(* Logix 5000 AddOnInstructionDefinition export ME_AOI_546xx_E02; software revision 20.05 *)

TYPE ME_IOL_PORT_32B :   // 32 Reserved IOL Bytes for IN & OUT
STRUCT
   in_data : SINT[32];
   out_data : SINT[32];
END_STRUCT
END_TYPE

TYPE ME_UDT_546xx_E02_In :   // 546xx Input Assembly
STRUCT
   Digital_Inputs : SINT[2];
   DI_Qualifier : SINT[2];
   DO_Qualifier : SINT[2];
   System_Status : ME_546xx_System_Status;
   Diagnostic_1 : ME_Diag_546xx;
   Diagnostic_2 : ME_Diag_546xx;
   Diagnostic_3 : ME_Diag_546xx;
   Diagnostic_4 : ME_Diag_546xx;
   Diagnostic_5 : ME_Diag_546xx;
   Diagnostic_6 : ME_Diag_546xx;
   Diagnostic_7 : ME_Diag_546xx;
   Diagnostic_8 : ME_Diag_546xx;
   IOL_PortX0_Status : ME_IOL_Port_X_Status_546xx;
   IOL_PortX1_Status : ME_IOL_Port_X_Status_546xx;
   IOL_PortX2_Status : ME_IOL_Port_X_Status_546xx;
   IOL_PortX3_Status : ME_IOL_Port_X_Status_546xx;
   IOL_PortX4_Status : ME_IOL_Port_X_Status_546xx;
   IOL_PortX5_Status : ME_IOL_Port_X_Status_546xx;
   IOL_PortX6_Status : ME_IOL_Port_X_Status_546xx;
   IOL_PortX7_Status : ME_IOL_Port_X_Status_546xx;
END_STRUCT
END_TYPE

TYPE ME_546xx_System_Status :   // Block Diagnostic Status
STRUCT
   Under_Voltage_Bus_Sensor_Supply : BOOL;
   Under_Voltage_Actuator_Supply : BOOL;
   No_Actuator_Supply : BOOL;
   External_Error : BOOL;
   Channel_Has_A_Sensor_Short_Circuit : BOOL;
   Channel_Has_An_Actuator_Short_Circuit : BOOL;
   Channel_Has_An_Actuator_Warning : BOOL;
   At_Least_One_Analog_Channel_Has_An_Error : BOOL;
   Internal_Communication_Error : BOOL;
   At_Least_One_IO_Link_Channel_Has_an_Erro : BOOL;
   Over_Voltage_Bus_Sensor_Supply : BOOL;
   Over_Voltage_Actuator_ASupply : BOOL;
   IO_Link_Channel_Has_A_Wire_Break : BOOL;
END_STRUCT
END_TYPE

TYPE ME_UDT_546xx_E02_Out :   // 546xx Output Assembly
STRUCT
   Digital_Outputs : SINT[2];
   Acknowledge : SINT[2];
END_STRUCT
END_TYPE

TYPE ME_Diag_546xx :   // Diagnostic Buffer for 546xx Modules
STRUCT
   IP : SINT;   // Last Octet of IP
   Identification : SINT;   // 0 = Default, 40h = IOL Master, 41h = IOL Device, 42h = Murr IOLD
   Channel_number : SINT;   // Digital Diag = Pin/Port IOL Diag = IOL Channel
   Error_Code_1 : SINT;   // Global Error Code or IOL LSB
   Error_Code_2 : SINT;   // Specific Error Code or IOL MSB
   Status : BOOL;   // 0 = Inactive, 1 = Active
   Severity : SINT;   // 1 = Minor, 2 = Major, 3 = Info
   Count : SINT;
END_STRUCT
END_TYPE

TYPE ME_UDT_546xx_E02 :   // Setup for EDS - E02 DIO + STATUS + DIAG
STRUCT
   I : ME_UDT_546xx_E02_In;
   O : ME_UDT_546xx_E02_Out;
END_STRUCT
END_TYPE

TYPE ME_IOL_Port_X_Status_546xx :   // Status of the IO-Link Device
STRUCT
   DevCom : BOOL;   // Pre-Operate or Operate Mode
   DevErr : BOOL;   // IOL Device Error or Warning
   PQ : BOOL;   // Valid Process Data Exchanged between Device & Master
   IOLD_Vendor_ID : SINT[2];   // Vendor ID of IO-Link Device
   IOLD_Device_ID : SINT[4];   // Device IP of IO-Link Device
END_STRUCT
END_TYPE

ADD_ON_INSTRUCTION ME_AOI_546xx_E02   (* revision 0.1 *)
VAR_IN_OUT
   Raw_546xx_Input : SINT[394]; {required}
   Raw_546xx_Output : SINT[259]; {required}
   Mapped_546xx_Communication_Data : ME_UDT_546xx_E02; {required}
   IO_Link_Port_X0 : ME_IOL_PORT_32B; {required}
        .I.DATA.0   // Input Port 0 Pin 4
        .I.DATA.1   // Input Port 0 Pin 2
        .I.DATA.2   // Input Port 1 Pin 4
        .I.DATA.3   // Input Port 1 Pin 2
        .I.DATA.4   // Input Port 2 Pin 4
        .I.DATA.5   // Input Port 2 Pin 2
        .I.DATA.6   // Input Port 3 Pin 4
        .I.DATA.7   // Input Port 3 Pin 2
        .I.DATA.8   // Input Port 4 Pin 4
        .I.DATA.9   // Input Port 4 Pin 2
        .I.DATA.10   // Input Port 5 Pin 4
        .I.DATA.11   // Input Port 5 Pin 2
        .I.DATA.12   // Input Port 6 Pin 4
        .I.DATA.13   // Input Port 6 Pin 2
        .I.DATA.14   // Input Port 7 Pin 4
        .I.DATA.15   // Input Port 7 Pin 2
        .I.OVERLOAD.0   // Port 0 Pin 4 Output Overload Status
        .I.OVERLOAD.1   // Port 0 Pin 2 Output Overload Status
        .I.OVERLOAD.2   // Port 1 Pin 4 Output Overload Status
        .I.OVERLOAD.3   // Port 1 Pin 2 Output Overload Status
        .I.OVERLOAD.4   // Port 2 Pin 4 Output Overload Status
        .I.OVERLOAD.5   // Port 2 Pin 2 Output Overload Status
        .I.OVERLOAD.6   // Port 3 Pin 4 Output Overload Status
        .I.OVERLOAD.7   // Port 3 Pin 2 Output Overload Status
        .I.OVERLOAD.8   // Port 4 Pin 4 Output Overload Status
        .I.OVERLOAD.9   // Port 4 Pin 2 Output Overload Status
        .I.OVERLOAD.10   // Port 5 Pin 4 Output Overload Status
        .I.OVERLOAD.11   // Port 5 Pin 2 Output Overload Status
        .I.OVERLOAD.12   // Port 6 Pin 4 Output Overload Status
        .I.OVERLOAD.13   // Port 6 Pin 2 Output Overload Status
        .I.OVERLOAD.14   // Port 7 Pin 4 Output Overload Status
        .I.OVERLOAD.15   // Port 7 Pin 2 Output Overload Status
        .I.PORT_1_DEVICE_CONNECTED   // Port 1 I/O Link Device Connected
        .I.PORT_1_IO_LINK_STATUS   // Port 1 In I/O Link Mode
        .I.PORT_1_VALIDATION_FAILED   // Port 1 I/O Link Device Configuration Mismatch
        .I.PORT_2_DEVICE_CONNECTED   // Port 2 I/O Link Device Connected
        .I.PORT_2_IO_LINK_STATUS   // Port 2 In I/O Link Mode
        .I.PORT_2_VALIDATION_FAILED   // Port 2 I/O Link Device Configuration Mismatch
        .I.PORT_3_DEVICE_CONNECTED   // Port 3 I/O Link Device Connected
        .I.PORT_3_IO_LINK_STATUS   // Port 3 In I/O Link Mode
        .I.PORT_3_VALIDATION_FAILED   // Port 3 I/O Link Device Configuration Mismatch
        .I.PORT_4_DEVICE_CONNECTED   // Port 4 I/O Link Device Connected
        .I.PORT_4_IO_LINK_STATUS   // Port 4 In I/O Link Mode
        .I.PORT_4_VALIDATION_FAILED   // Port 4 I/O Link Device Configuration Mismatch
        .I.SHORT_CIRCUIT.0   // Port 0 Pin 4 Short Circuit
        .I.SHORT_CIRCUIT.1   // Port 0 Pin 2 Short Circuit
        .I.SHORT_CIRCUIT.2   // Port 1 Pin 4 Short Circuit
        .I.SHORT_CIRCUIT.3   // Port 1 Pin 2 Short Circuit
        .I.SHORT_CIRCUIT.4   // Port 2 Pin 4 Short Circuit
        .I.SHORT_CIRCUIT.5   // Port 2 Pin 2 Short Circuit
        .I.SHORT_CIRCUIT.6   // Port 3 Pin 4 Short Circuit
        .I.SHORT_CIRCUIT.7   // Port 3 Pin 2 Short Circuit
        .I.SHORT_CIRCUIT.8   // Port 4 Pin 4 Short Circuit
        .I.SHORT_CIRCUIT.9   // Port 4 Pin 2 Short Circuit
        .I.SHORT_CIRCUIT.10   // Port 5 Pin 4 Short Circuit
        .I.SHORT_CIRCUIT.11   // Port 5 Pin 2 Short Circuit
        .I.SHORT_CIRCUIT.12   // Port 6 Pin 4 Short Circuit
        .I.SHORT_CIRCUIT.13   // Port 6 Pin 2 Short Circuit
        .I.SHORT_CIRCUIT.14   // Port 7 Pin 4 Short Circuit
        .I.SHORT_CIRCUIT.15   // Port 7 Pin 2 Short Circuit
        .I.UA_FAULT   // Output Power from Aux Power cable Under Voltage
        .I.US_FAULT   // Module Power from IO-Link Communication Cable Under Voltage
        .O.DATA.0   // Output Port 0 Pin 4
        .O.DATA.1   // Output Port 0 Pin 2
        .O.DATA.2   // Output Port 1 Pin 4
        .O.DATA.3   // Output Port 1 Pin 2
        .O.DATA.4   // Output Port 2 Pin 4
        .O.DATA.5   // Output Port 2 Pin 2
        .O.DATA.6   // Output Port 3 Pin 4
        .O.DATA.7   // Output Port 3 Pin 2
        .O.DATA.8   // Output Port 4 Pin 4
        .O.DATA.9   // Output Port 4 Pin 2
        .O.DATA.10   // Output Port 5 Pin 4
        .O.DATA.11   // Output Port 5 Pin 2
        .O.DATA.12   // Output Port 6 Pin 4
        .O.DATA.13   // Output Port 6 Pin 2
        .O.DATA.14   // Output Port 7 Pin 4
        .O.DATA.15   // Output Port 7 Pin 2
        .O.DISPLAY_GREEN   // Green LED On
        .O.DISPLAY_LOCK   // Display Lock PLC Lock
        .O.DISPLAY_RED   // Red LED On
        .O.RESTART.0   // Port 0 Pin 4 Output Restart
        .O.RESTART.1   // Port 0 Pin 2 Output Restart
        .O.RESTART.2   // Port 1 Pin 4 Output Restart
        .O.RESTART.3   // Port 1 Pin 2 Output Restart
        .O.RESTART.4   // Port 2 Pin 4 Output Restart
        .O.RESTART.5   // Port 2 Pin 2 Output Restart
        .O.RESTART.6   // Port 3 Pin 4 Output Restart
        .O.RESTART.7   // Port 3 Pin 2 Output Restart
        .O.RESTART.8   // Port 4 Pin 4 Output Restart
        .O.RESTART.9   // Port 4 Pin 2 Output Restart
        .O.RESTART.10   // Port 5 Pin 4 Output Restart
        .O.RESTART.11   // Port 5 Pin 2 Output Restart
        .O.RESTART.12   // Port 6 Pin 4 Output Restart
        .O.RESTART.13   // Port 6 Pin 2 Output Restart
        .O.RESTART.14   // Port 7 Pin 4 Output Restart
        .O.RESTART.15   // Port 7 Pin 2 Output Restart
   IO_Link_Port_X1 : ME_IOL_PORT_32B; {required}
   IO_Link_Port_X2 : ME_IOL_PORT_32B; {required}
   IO_Link_Port_X3 : ME_IOL_PORT_32B; {required}
   IO_Link_Port_X4 : ME_IOL_PORT_32B; {required}
   IO_Link_Port_X5 : ME_IOL_PORT_32B; {required}
   IO_Link_Port_X6 : ME_IOL_PORT_32B; {required}
   IO_Link_Port_X7 : ME_IOL_PORT_32B; {required}
END_VAR

ROUTINE Logic   (* ladder *)
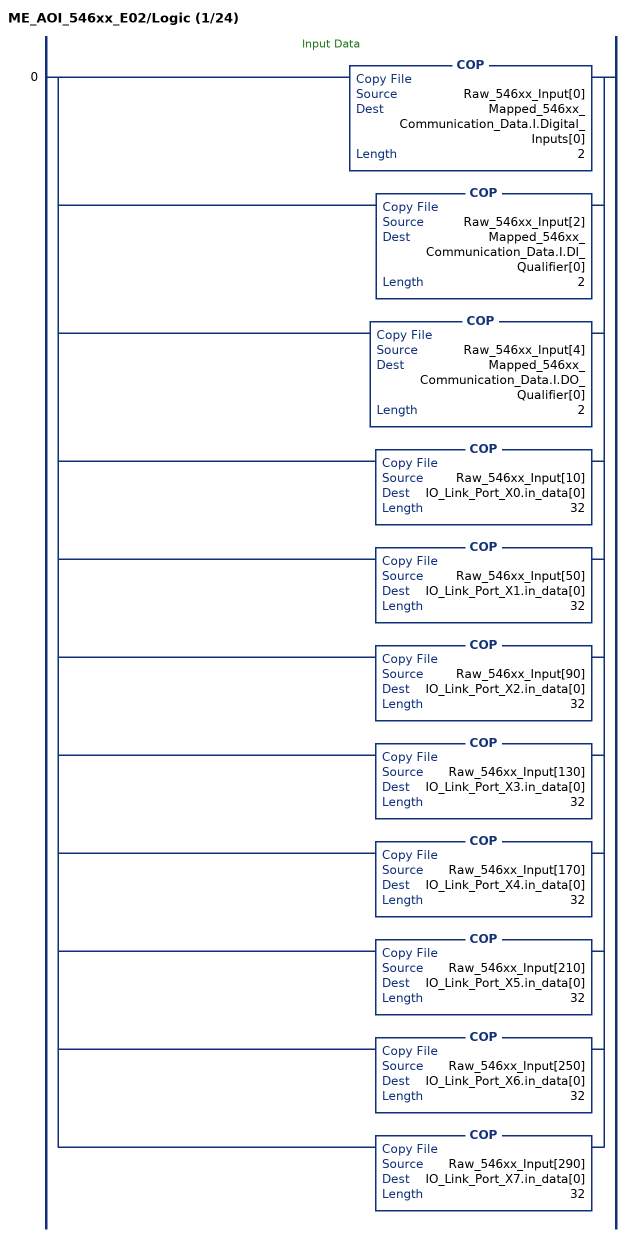
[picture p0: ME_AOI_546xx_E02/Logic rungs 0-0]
   // Input Data
   0: [COP(Raw_546xx_Input[0],Mapped_546xx_Communication_Data.I.Digital_Inputs[0],2) ,COP(Raw_546xx_Input[2],Mapped_546xx_Communication_Data.I.DI_Qualifier[0],2) ,COP(Raw_546xx_Input[4],Mapped_546xx_Communication_Data.I.DO_Qualifier[0],2) ,COP(Raw_546xx_Input[10],IO_Link_Port_X0.in_data[0],32) ,COP(Raw_546xx_Input[50],IO_Link_Port_X1.in_data[0],32) ,COP(Raw_546xx_Input[90],IO_Link_Port_X2.in_data[0],32) ,COP(Raw_546xx_Input[130],IO_Link_Port_X3.in_data[0],32) ,COP(Raw_546xx_Input[170],IO_Link_Port_X4.in_data[0],32) ,COP(Raw_546xx_Input[210],IO_Link_Port_X5.in_data[0],32) ,COP(Raw_546xx_Input[250],IO_Link_Port_X6.in_data[0],32) ,COP(Raw_546xx_Input[290],IO_Link_Port_X7.in_data[0],32) ];
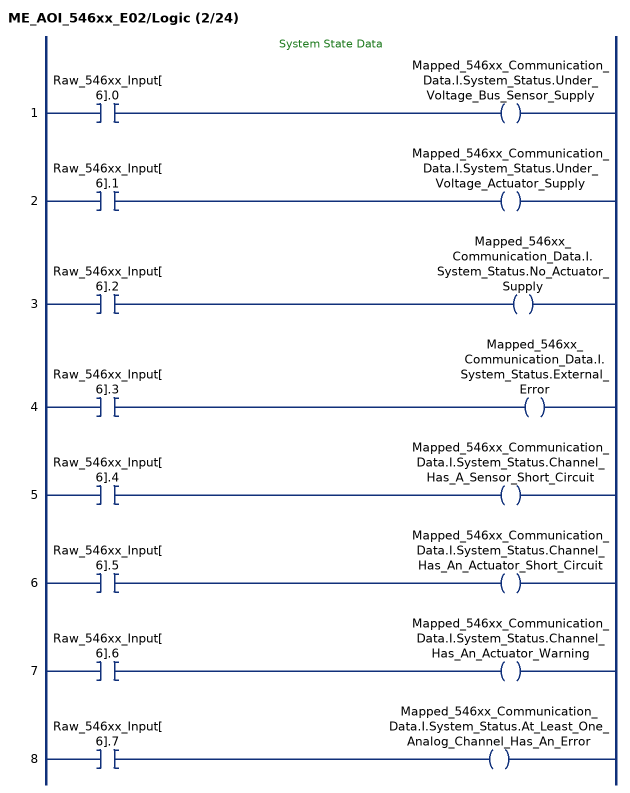
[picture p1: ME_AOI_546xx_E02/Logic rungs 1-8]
   // System State Data
   1: XIC(Raw_546xx_Input[6].0)OTE(Mapped_546xx_Communication_Data.I.System_Status.Under_Voltage_Bus_Sensor_Supply);
   2: XIC(Raw_546xx_Input[6].1)OTE(Mapped_546xx_Communication_Data.I.System_Status.Under_Voltage_Actuator_Supply);
   3: XIC(Raw_546xx_Input[6].2)OTE(Mapped_546xx_Communication_Data.I.System_Status.No_Actuator_Supply);
   4: XIC(Raw_546xx_Input[6].3)OTE(Mapped_546xx_Communication_Data.I.System_Status.External_Error);
   5: XIC(Raw_546xx_Input[6].4)OTE(Mapped_546xx_Communication_Data.I.System_Status.Channel_Has_A_Sensor_Short_Circuit);
   6: XIC(Raw_546xx_Input[6].5)OTE(Mapped_546xx_Communication_Data.I.System_Status.Channel_Has_An_Actuator_Short_Circuit);
   7: XIC(Raw_546xx_Input[6].6)OTE(Mapped_546xx_Communication_Data.I.System_Status.Channel_Has_An_Actuator_Warning);
   8: XIC(Raw_546xx_Input[6].7)OTE(Mapped_546xx_Communication_Data.I.System_Status.At_Least_One_Analog_Channel_Has_An_Error);
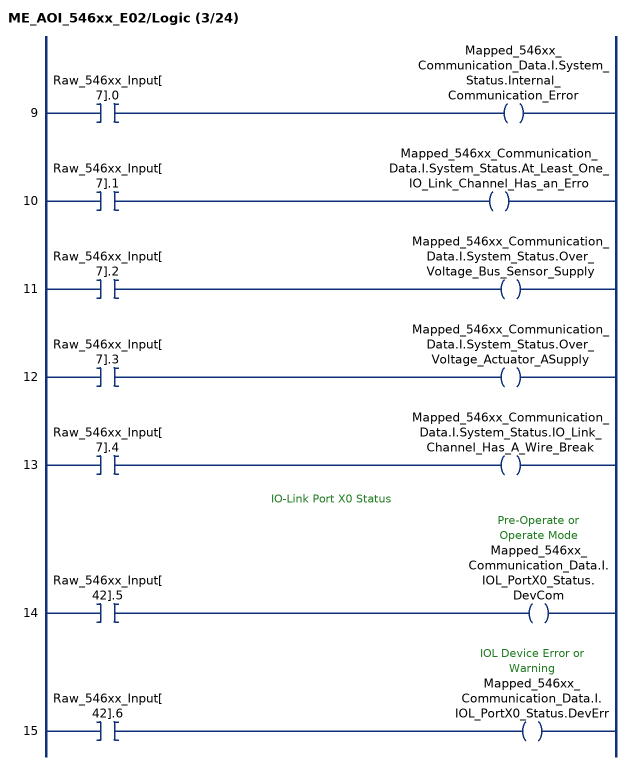
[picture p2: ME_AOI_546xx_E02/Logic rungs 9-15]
   9: XIC(Raw_546xx_Input[7].0)OTE(Mapped_546xx_Communication_Data.I.System_Status.Internal_Communication_Error);
   10: XIC(Raw_546xx_Input[7].1)OTE(Mapped_546xx_Communication_Data.I.System_Status.At_Least_One_IO_Link_Channel_Has_an_Erro);
   11: XIC(Raw_546xx_Input[7].2)OTE(Mapped_546xx_Communication_Data.I.System_Status.Over_Voltage_Bus_Sensor_Supply);
   12: XIC(Raw_546xx_Input[7].3)OTE(Mapped_546xx_Communication_Data.I.System_Status.Over_Voltage_Actuator_ASupply);
   13: XIC(Raw_546xx_Input[7].4)OTE(Mapped_546xx_Communication_Data.I.System_Status.IO_Link_Channel_Has_A_Wire_Break);
   // IO-Link Port X0 Status
   14: XIC(Raw_546xx_Input[42].5)OTE(Mapped_546xx_Communication_Data.I.IOL_PortX0_Status.DevCom);
   15: XIC(Raw_546xx_Input[42].6)OTE(Mapped_546xx_Communication_Data.I.IOL_PortX0_Status.DevErr);
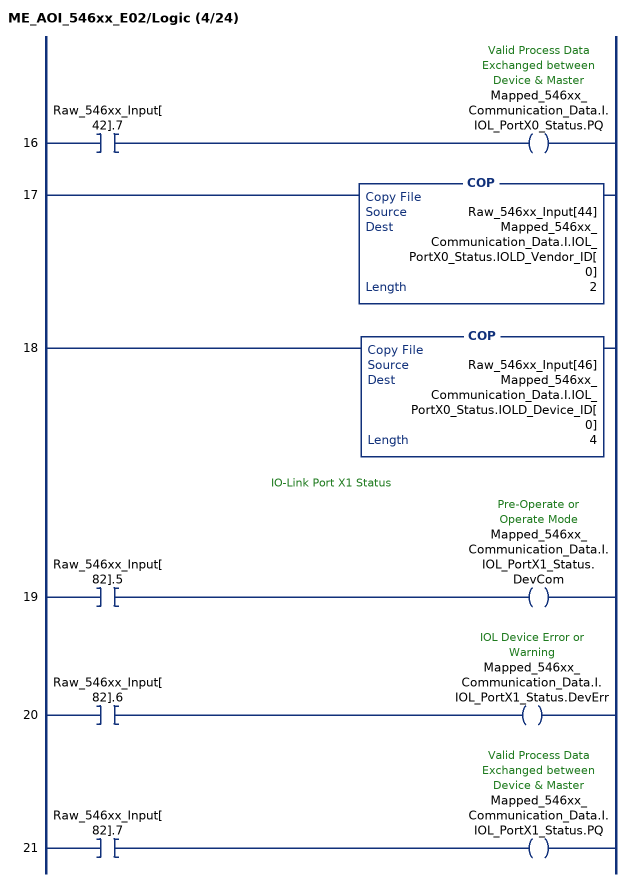
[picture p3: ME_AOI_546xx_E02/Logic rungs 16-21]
   16: XIC(Raw_546xx_Input[42].7)OTE(Mapped_546xx_Communication_Data.I.IOL_PortX0_Status.PQ);
   17: COP(Raw_546xx_Input[44],Mapped_546xx_Communication_Data.I.IOL_PortX0_Status.IOLD_Vendor_ID[0],2);
   18: COP(Raw_546xx_Input[46],Mapped_546xx_Communication_Data.I.IOL_PortX0_Status.IOLD_Device_ID[0],4);
   // IO-Link Port X1 Status
   19: XIC(Raw_546xx_Input[82].5)OTE(Mapped_546xx_Communication_Data.I.IOL_PortX1_Status.DevCom);
   20: XIC(Raw_546xx_Input[82].6)OTE(Mapped_546xx_Communication_Data.I.IOL_PortX1_Status.DevErr);
   21: XIC(Raw_546xx_Input[82].7)OTE(Mapped_546xx_Communication_Data.I.IOL_PortX1_Status.PQ);
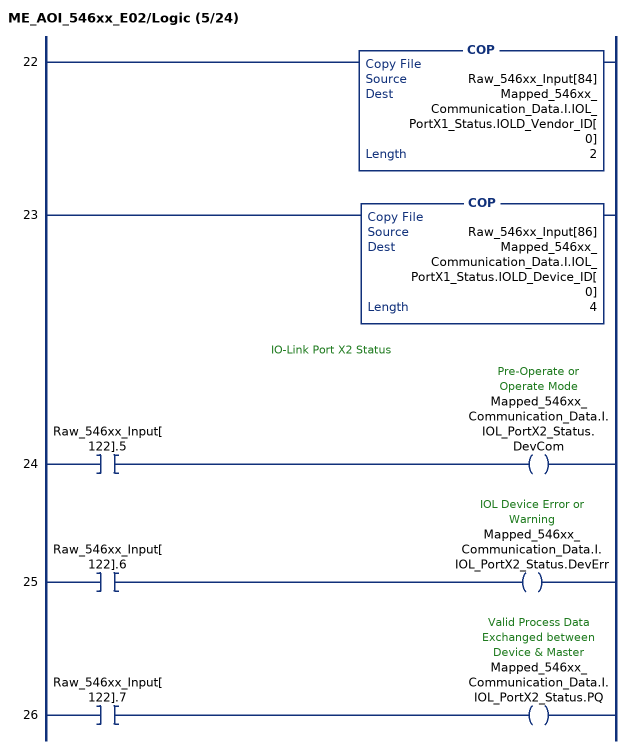
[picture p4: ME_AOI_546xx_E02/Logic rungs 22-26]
   22: COP(Raw_546xx_Input[84],Mapped_546xx_Communication_Data.I.IOL_PortX1_Status.IOLD_Vendor_ID[0],2);
   23: COP(Raw_546xx_Input[86],Mapped_546xx_Communication_Data.I.IOL_PortX1_Status.IOLD_Device_ID[0],4);
   // IO-Link Port X2 Status
   24: XIC(Raw_546xx_Input[122].5)OTE(Mapped_546xx_Communication_Data.I.IOL_PortX2_Status.DevCom);
   25: XIC(Raw_546xx_Input[122].6)OTE(Mapped_546xx_Communication_Data.I.IOL_PortX2_Status.DevErr);
   26: XIC(Raw_546xx_Input[122].7)OTE(Mapped_546xx_Communication_Data.I.IOL_PortX2_Status.PQ);
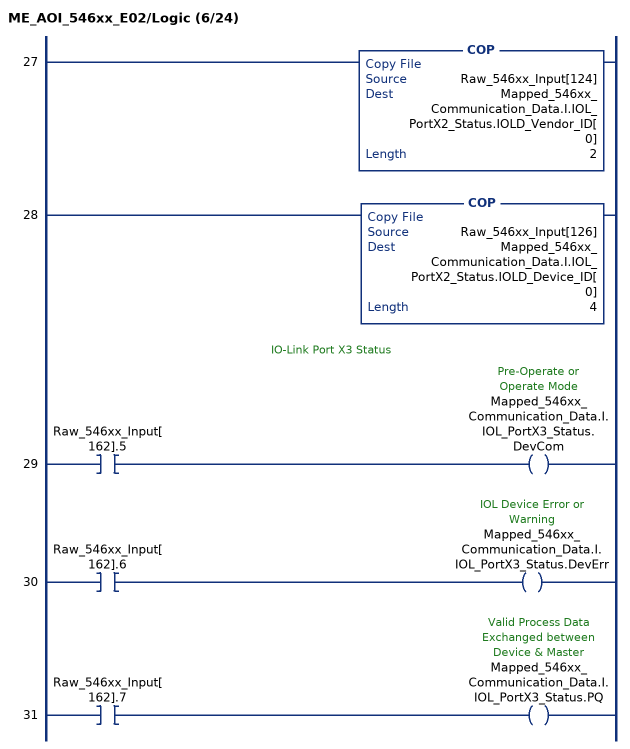
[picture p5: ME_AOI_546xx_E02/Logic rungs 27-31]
   27: COP(Raw_546xx_Input[124],Mapped_546xx_Communication_Data.I.IOL_PortX2_Status.IOLD_Vendor_ID[0],2);
   28: COP(Raw_546xx_Input[126],Mapped_546xx_Communication_Data.I.IOL_PortX2_Status.IOLD_Device_ID[0],4);
   // IO-Link Port X3 Status
   29: XIC(Raw_546xx_Input[162].5)OTE(Mapped_546xx_Communication_Data.I.IOL_PortX3_Status.DevCom);
   30: XIC(Raw_546xx_Input[162].6)OTE(Mapped_546xx_Communication_Data.I.IOL_PortX3_Status.DevErr);
   31: XIC(Raw_546xx_Input[162].7)OTE(Mapped_546xx_Communication_Data.I.IOL_PortX3_Status.PQ);
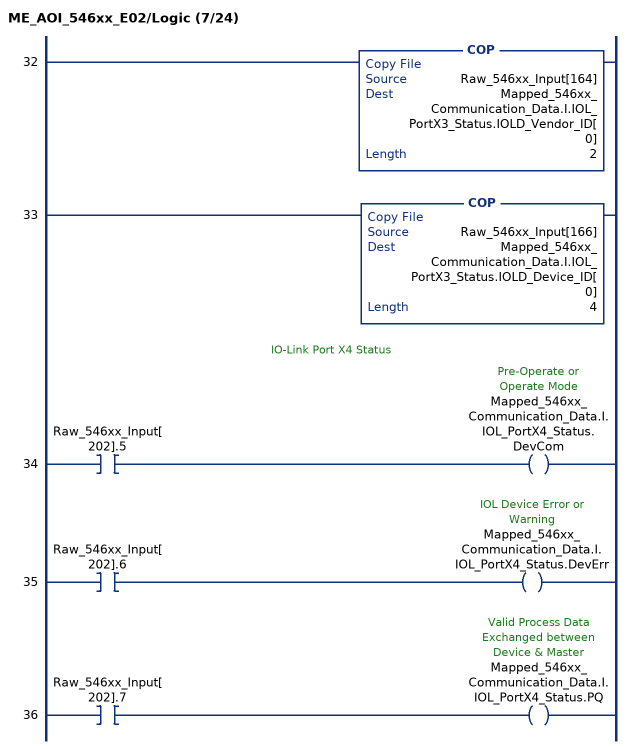
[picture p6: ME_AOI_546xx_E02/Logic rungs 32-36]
   32: COP(Raw_546xx_Input[164],Mapped_546xx_Communication_Data.I.IOL_PortX3_Status.IOLD_Vendor_ID[0],2);
   33: COP(Raw_546xx_Input[166],Mapped_546xx_Communication_Data.I.IOL_PortX3_Status.IOLD_Device_ID[0],4);
   // IO-Link Port X4 Status
   34: XIC(Raw_546xx_Input[202].5)OTE(Mapped_546xx_Communication_Data.I.IOL_PortX4_Status.DevCom);
   35: XIC(Raw_546xx_Input[202].6)OTE(Mapped_546xx_Communication_Data.I.IOL_PortX4_Status.DevErr);
   36: XIC(Raw_546xx_Input[202].7)OTE(Mapped_546xx_Communication_Data.I.IOL_PortX4_Status.PQ);
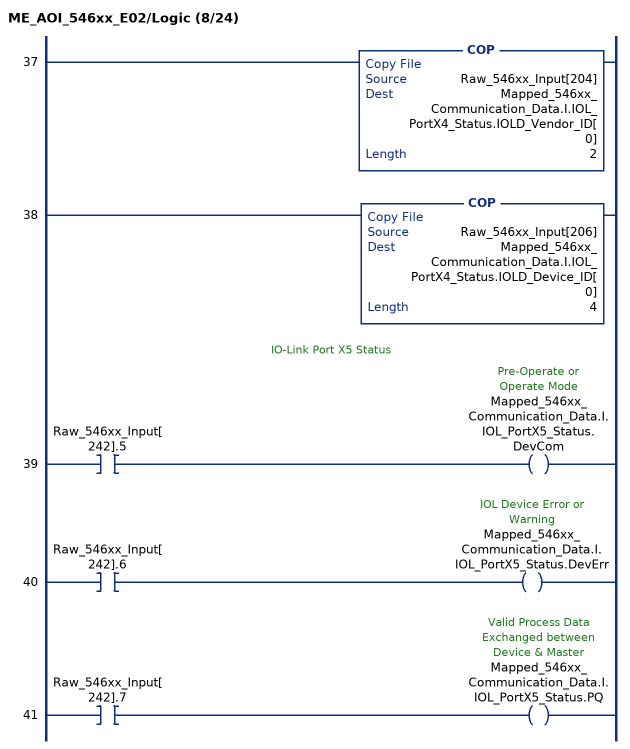
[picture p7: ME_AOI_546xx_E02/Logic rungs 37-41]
   37: COP(Raw_546xx_Input[204],Mapped_546xx_Communication_Data.I.IOL_PortX4_Status.IOLD_Vendor_ID[0],2);
   38: COP(Raw_546xx_Input[206],Mapped_546xx_Communication_Data.I.IOL_PortX4_Status.IOLD_Device_ID[0],4);
   // IO-Link Port X5 Status
   39: XIC(Raw_546xx_Input[242].5)OTE(Mapped_546xx_Communication_Data.I.IOL_PortX5_Status.DevCom);
   40: XIC(Raw_546xx_Input[242].6)OTE(Mapped_546xx_Communication_Data.I.IOL_PortX5_Status.DevErr);
   41: XIC(Raw_546xx_Input[242].7)OTE(Mapped_546xx_Communication_Data.I.IOL_PortX5_Status.PQ);
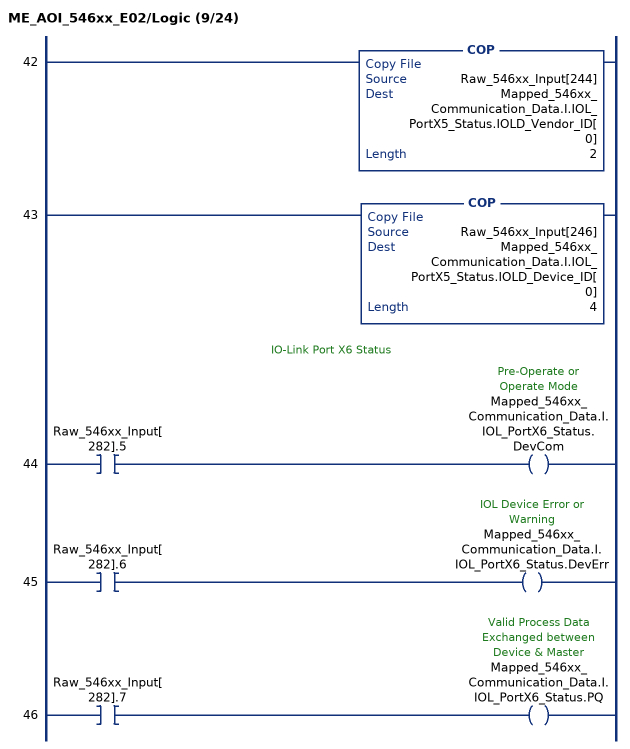
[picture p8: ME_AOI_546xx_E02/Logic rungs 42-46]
   42: COP(Raw_546xx_Input[244],Mapped_546xx_Communication_Data.I.IOL_PortX5_Status.IOLD_Vendor_ID[0],2);
   43: COP(Raw_546xx_Input[246],Mapped_546xx_Communication_Data.I.IOL_PortX5_Status.IOLD_Device_ID[0],4);
   // IO-Link Port X6 Status
   44: XIC(Raw_546xx_Input[282].5)OTE(Mapped_546xx_Communication_Data.I.IOL_PortX6_Status.DevCom);
   45: XIC(Raw_546xx_Input[282].6)OTE(Mapped_546xx_Communication_Data.I.IOL_PortX6_Status.DevErr);
   46: XIC(Raw_546xx_Input[282].7)OTE(Mapped_546xx_Communication_Data.I.IOL_PortX6_Status.PQ);
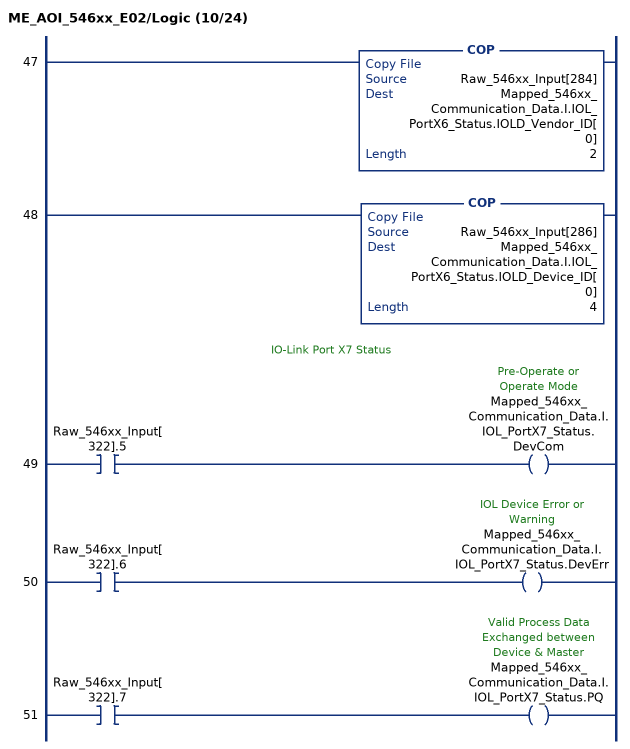
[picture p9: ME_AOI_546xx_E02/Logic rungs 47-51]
   47: COP(Raw_546xx_Input[284],Mapped_546xx_Communication_Data.I.IOL_PortX6_Status.IOLD_Vendor_ID[0],2);
   48: COP(Raw_546xx_Input[286],Mapped_546xx_Communication_Data.I.IOL_PortX6_Status.IOLD_Device_ID[0],4);
   // IO-Link Port X7 Status
   49: XIC(Raw_546xx_Input[322].5)OTE(Mapped_546xx_Communication_Data.I.IOL_PortX7_Status.DevCom);
   50: XIC(Raw_546xx_Input[322].6)OTE(Mapped_546xx_Communication_Data.I.IOL_PortX7_Status.DevErr);
   51: XIC(Raw_546xx_Input[322].7)OTE(Mapped_546xx_Communication_Data.I.IOL_PortX7_Status.PQ);
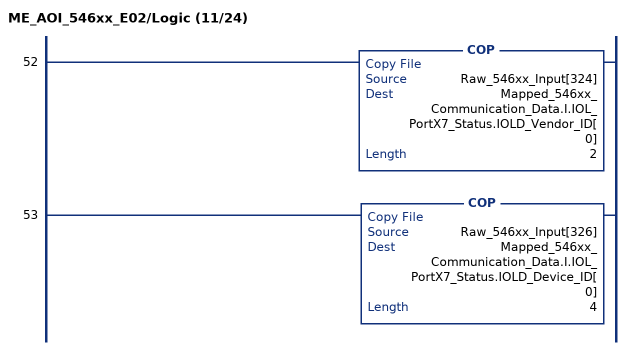
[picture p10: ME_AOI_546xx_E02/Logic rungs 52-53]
   52: COP(Raw_546xx_Input[324],Mapped_546xx_Communication_Data.I.IOL_PortX7_Status.IOLD_Vendor_ID[0],2);
   53: COP(Raw_546xx_Input[326],Mapped_546xx_Communication_Data.I.IOL_PortX7_Status.IOLD_Device_ID[0],4);
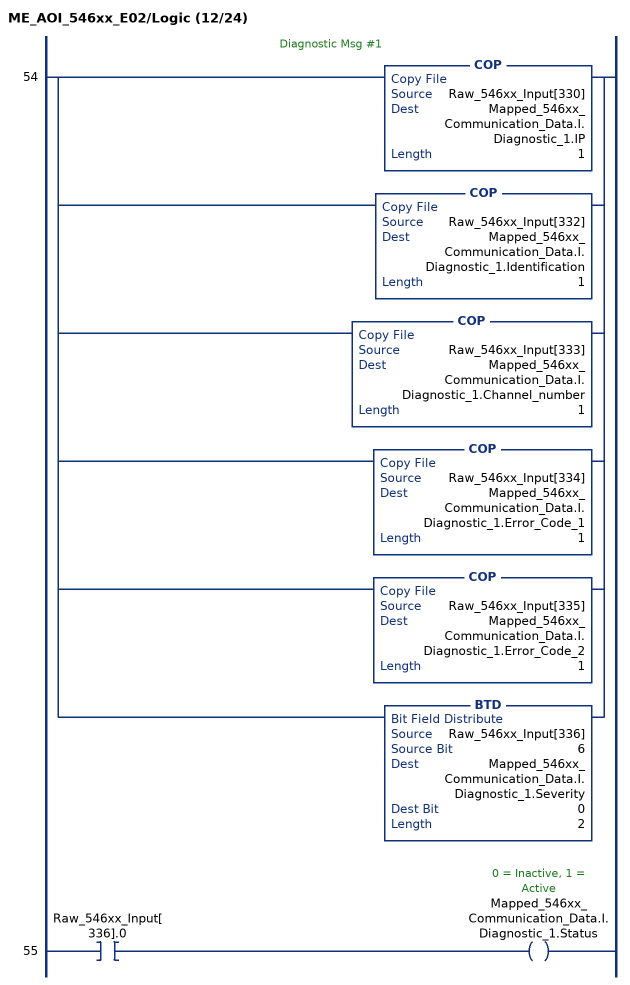
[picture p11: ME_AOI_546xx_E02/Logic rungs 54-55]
   // Diagnostic Msg #1
   54: [COP(Raw_546xx_Input[330],Mapped_546xx_Communication_Data.I.Diagnostic_1.IP,1) ,COP(Raw_546xx_Input[332],Mapped_546xx_Communication_Data.I.Diagnostic_1.Identification,1) ,COP(Raw_546xx_Input[333],Mapped_546xx_Communication_Data.I.Diagnostic_1.Channel_number,1) ,COP(Raw_546xx_Input[334],Mapped_546xx_Communication_Data.I.Diagnostic_1.Error_Code_1,1) ,COP(Raw_546xx_Input[335],Mapped_546xx_Communication_Data.I.Diagnostic_1.Error_Code_2,1) ,BTD(Raw_546xx_Input[336],6,Mapped_546xx_Communication_Data.I.Diagnostic_1.Severity,0,2) ];
   55: XIC(Raw_546xx_Input[336].0)OTE(Mapped_546xx_Communication_Data.I.Diagnostic_1.Status);
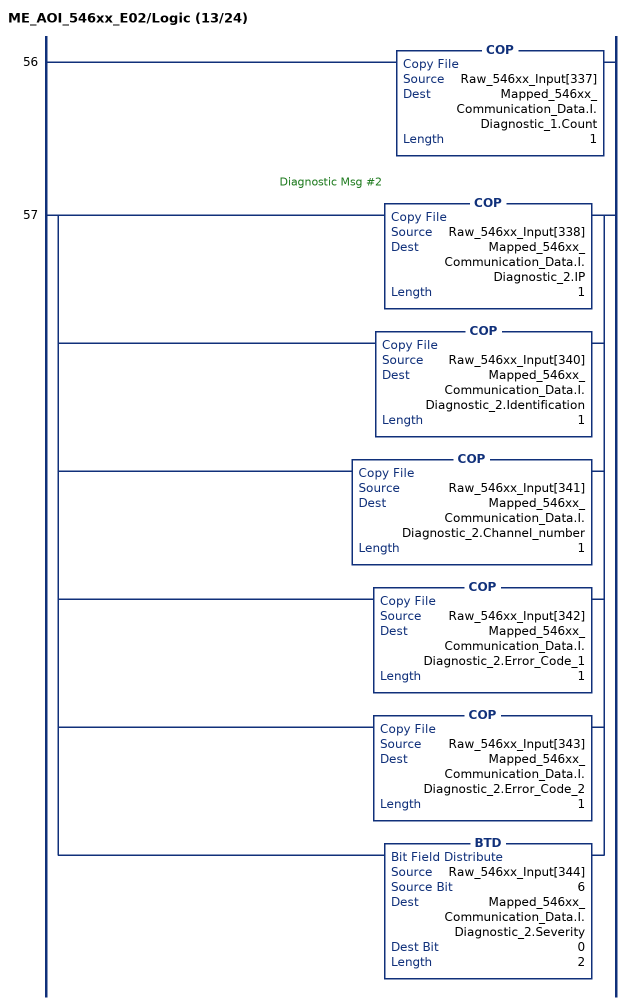
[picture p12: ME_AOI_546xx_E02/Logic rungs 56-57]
   56: COP(Raw_546xx_Input[337],Mapped_546xx_Communication_Data.I.Diagnostic_1.Count,1);
   // Diagnostic Msg #2
   57: [COP(Raw_546xx_Input[338],Mapped_546xx_Communication_Data.I.Diagnostic_2.IP,1) ,COP(Raw_546xx_Input[340],Mapped_546xx_Communication_Data.I.Diagnostic_2.Identification,1) ,COP(Raw_546xx_Input[341],Mapped_546xx_Communication_Data.I.Diagnostic_2.Channel_number,1) ,COP(Raw_546xx_Input[342],Mapped_546xx_Communication_Data.I.Diagnostic_2.Error_Code_1,1) ,COP(Raw_546xx_Input[343],Mapped_546xx_Communication_Data.I.Diagnostic_2.Error_Code_2,1) ,BTD(Raw_546xx_Input[344],6,Mapped_546xx_Communication_Data.I.Diagnostic_2.Severity,0,2) ];
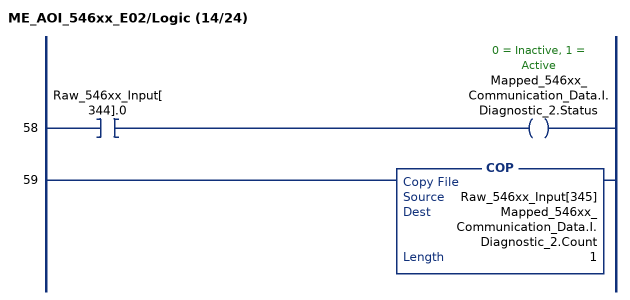
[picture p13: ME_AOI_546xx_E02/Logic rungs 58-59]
   58: XIC(Raw_546xx_Input[344].0)OTE(Mapped_546xx_Communication_Data.I.Diagnostic_2.Status);
   59: COP(Raw_546xx_Input[345],Mapped_546xx_Communication_Data.I.Diagnostic_2.Count,1);
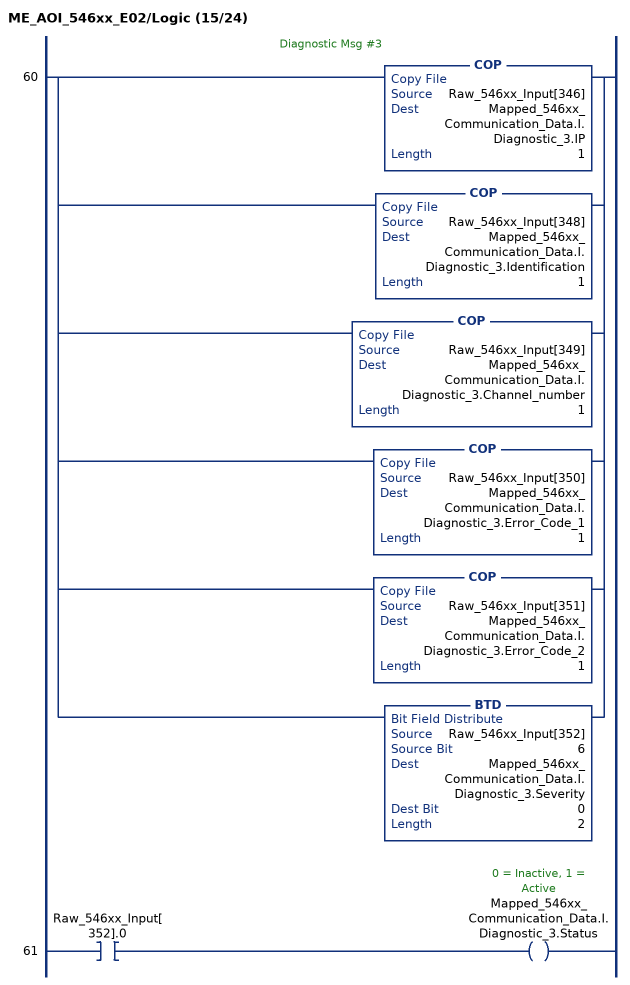
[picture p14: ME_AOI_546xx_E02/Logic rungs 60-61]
   // Diagnostic Msg #3
   60: [COP(Raw_546xx_Input[346],Mapped_546xx_Communication_Data.I.Diagnostic_3.IP,1) ,COP(Raw_546xx_Input[348],Mapped_546xx_Communication_Data.I.Diagnostic_3.Identification,1) ,COP(Raw_546xx_Input[349],Mapped_546xx_Communication_Data.I.Diagnostic_3.Channel_number,1) ,COP(Raw_546xx_Input[350],Mapped_546xx_Communication_Data.I.Diagnostic_3.Error_Code_1,1) ,COP(Raw_546xx_Input[351],Mapped_546xx_Communication_Data.I.Diagnostic_3.Error_Code_2,1) ,BTD(Raw_546xx_Input[352],6,Mapped_546xx_Communication_Data.I.Diagnostic_3.Severity,0,2) ];
   61: XIC(Raw_546xx_Input[352].0)OTE(Mapped_546xx_Communication_Data.I.Diagnostic_3.Status);
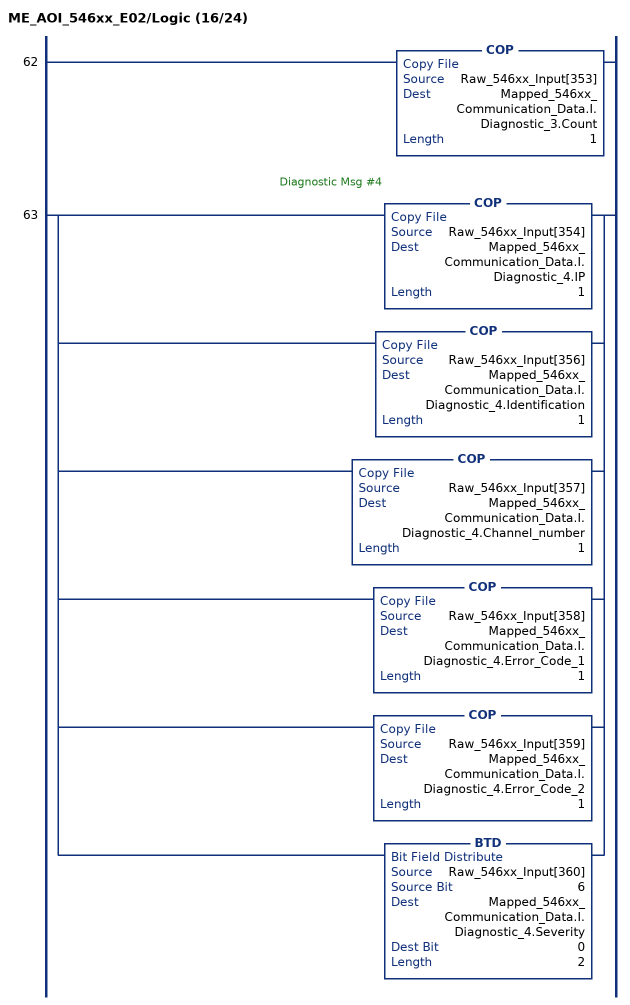
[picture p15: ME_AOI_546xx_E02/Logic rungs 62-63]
   62: COP(Raw_546xx_Input[353],Mapped_546xx_Communication_Data.I.Diagnostic_3.Count,1);
   // Diagnostic Msg #4
   63: [COP(Raw_546xx_Input[354],Mapped_546xx_Communication_Data.I.Diagnostic_4.IP,1) ,COP(Raw_546xx_Input[356],Mapped_546xx_Communication_Data.I.Diagnostic_4.Identification,1) ,COP(Raw_546xx_Input[357],Mapped_546xx_Communication_Data.I.Diagnostic_4.Channel_number,1) ,COP(Raw_546xx_Input[358],Mapped_546xx_Communication_Data.I.Diagnostic_4.Error_Code_1,1) ,COP(Raw_546xx_Input[359],Mapped_546xx_Communication_Data.I.Diagnostic_4.Error_Code_2,1) ,BTD(Raw_546xx_Input[360],6,Mapped_546xx_Communication_Data.I.Diagnostic_4.Severity,0,2) ];
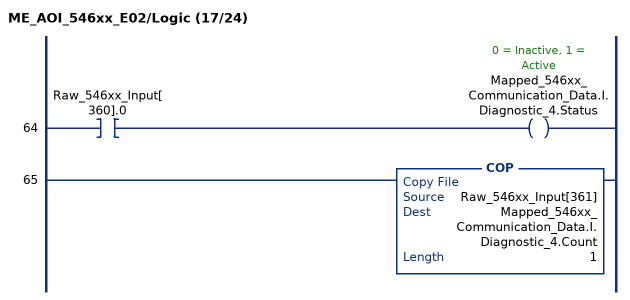
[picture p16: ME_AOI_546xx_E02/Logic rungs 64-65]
   64: XIC(Raw_546xx_Input[360].0)OTE(Mapped_546xx_Communication_Data.I.Diagnostic_4.Status);
   65: COP(Raw_546xx_Input[361],Mapped_546xx_Communication_Data.I.Diagnostic_4.Count,1);
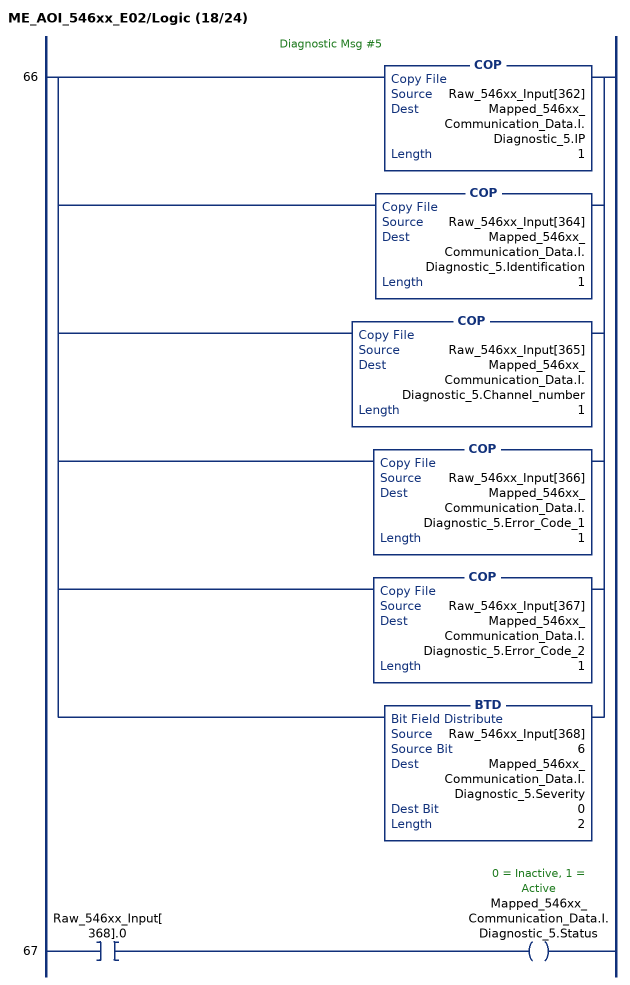
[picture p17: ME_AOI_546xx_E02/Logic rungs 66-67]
   // Diagnostic Msg #5
   66: [COP(Raw_546xx_Input[362],Mapped_546xx_Communication_Data.I.Diagnostic_5.IP,1) ,COP(Raw_546xx_Input[364],Mapped_546xx_Communication_Data.I.Diagnostic_5.Identification,1) ,COP(Raw_546xx_Input[365],Mapped_546xx_Communication_Data.I.Diagnostic_5.Channel_number,1) ,COP(Raw_546xx_Input[366],Mapped_546xx_Communication_Data.I.Diagnostic_5.Error_Code_1,1) ,COP(Raw_546xx_Input[367],Mapped_546xx_Communication_Data.I.Diagnostic_5.Error_Code_2,1) ,BTD(Raw_546xx_Input[368],6,Mapped_546xx_Communication_Data.I.Diagnostic_5.Severity,0,2) ];
   67: XIC(Raw_546xx_Input[368].0)OTE(Mapped_546xx_Communication_Data.I.Diagnostic_5.Status);
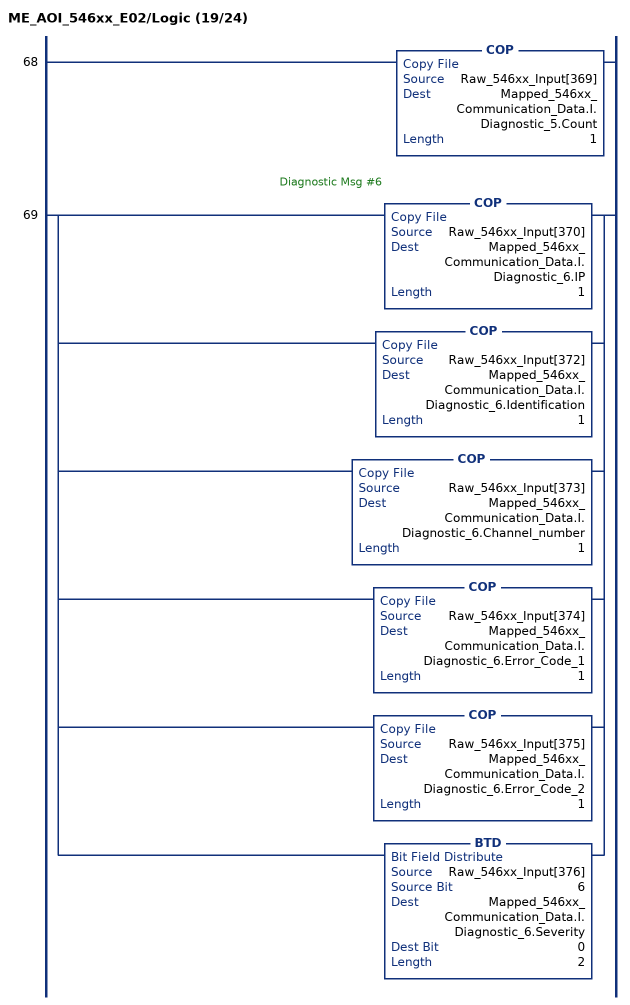
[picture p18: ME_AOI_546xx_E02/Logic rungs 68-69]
   68: COP(Raw_546xx_Input[369],Mapped_546xx_Communication_Data.I.Diagnostic_5.Count,1);
   // Diagnostic Msg #6
   69: [COP(Raw_546xx_Input[370],Mapped_546xx_Communication_Data.I.Diagnostic_6.IP,1) ,COP(Raw_546xx_Input[372],Mapped_546xx_Communication_Data.I.Diagnostic_6.Identification,1) ,COP(Raw_546xx_Input[373],Mapped_546xx_Communication_Data.I.Diagnostic_6.Channel_number,1) ,COP(Raw_546xx_Input[374],Mapped_546xx_Communication_Data.I.Diagnostic_6.Error_Code_1,1) ,COP(Raw_546xx_Input[375],Mapped_546xx_Communication_Data.I.Diagnostic_6.Error_Code_2,1) ,BTD(Raw_546xx_Input[376],6,Mapped_546xx_Communication_Data.I.Diagnostic_6.Severity,0,2) ];
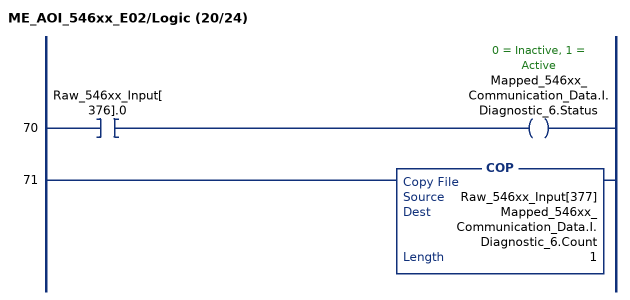
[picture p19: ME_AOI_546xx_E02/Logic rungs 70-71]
   70: XIC(Raw_546xx_Input[376].0)OTE(Mapped_546xx_Communication_Data.I.Diagnostic_6.Status);
   71: COP(Raw_546xx_Input[377],Mapped_546xx_Communication_Data.I.Diagnostic_6.Count,1);
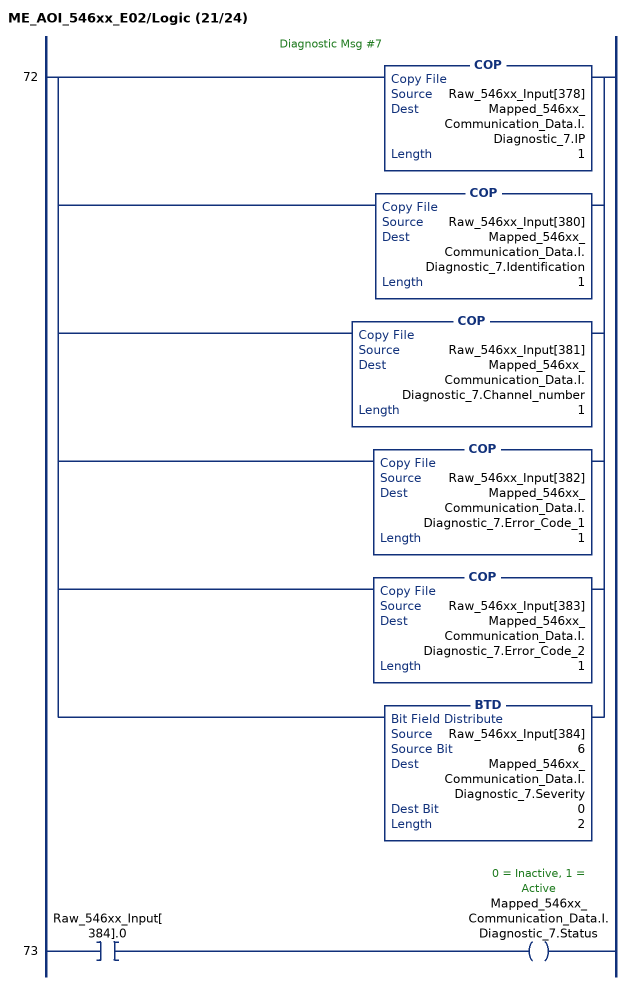
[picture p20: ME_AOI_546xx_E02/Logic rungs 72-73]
   // Diagnostic Msg #7
   72: [COP(Raw_546xx_Input[378],Mapped_546xx_Communication_Data.I.Diagnostic_7.IP,1) ,COP(Raw_546xx_Input[380],Mapped_546xx_Communication_Data.I.Diagnostic_7.Identification,1) ,COP(Raw_546xx_Input[381],Mapped_546xx_Communication_Data.I.Diagnostic_7.Channel_number,1) ,COP(Raw_546xx_Input[382],Mapped_546xx_Communication_Data.I.Diagnostic_7.Error_Code_1,1) ,COP(Raw_546xx_Input[383],Mapped_546xx_Communication_Data.I.Diagnostic_7.Error_Code_2,1) ,BTD(Raw_546xx_Input[384],6,Mapped_546xx_Communication_Data.I.Diagnostic_7.Severity,0,2) ];
   73: XIC(Raw_546xx_Input[384].0)OTE(Mapped_546xx_Communication_Data.I.Diagnostic_7.Status);
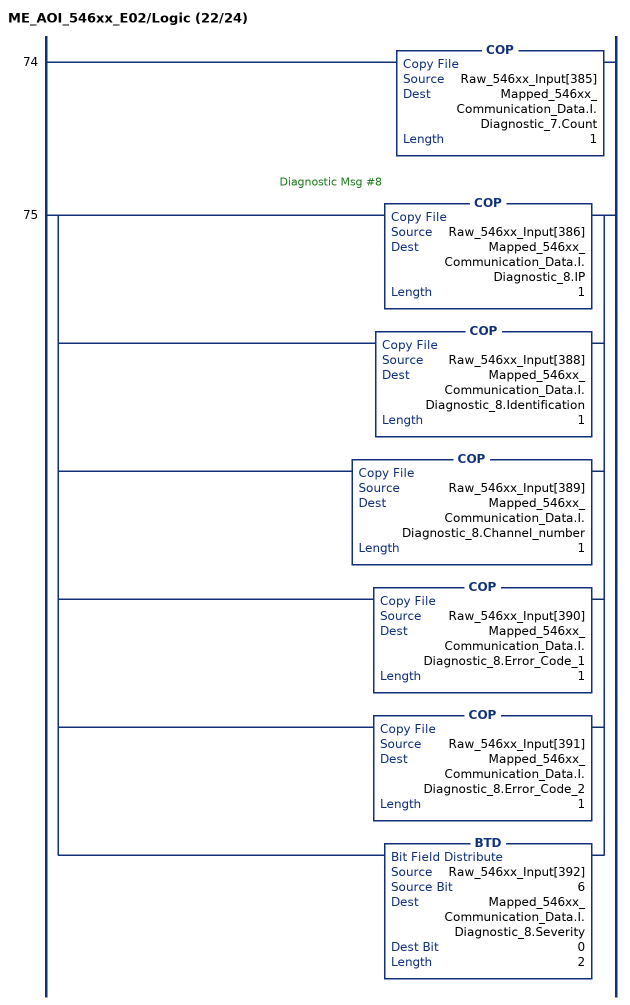
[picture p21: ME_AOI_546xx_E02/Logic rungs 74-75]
   74: COP(Raw_546xx_Input[385],Mapped_546xx_Communication_Data.I.Diagnostic_7.Count,1);
   // Diagnostic Msg #8
   75: [COP(Raw_546xx_Input[386],Mapped_546xx_Communication_Data.I.Diagnostic_8.IP,1) ,COP(Raw_546xx_Input[388],Mapped_546xx_Communication_Data.I.Diagnostic_8.Identification,1) ,COP(Raw_546xx_Input[389],Mapped_546xx_Communication_Data.I.Diagnostic_8.Channel_number,1) ,COP(Raw_546xx_Input[390],Mapped_546xx_Communication_Data.I.Diagnostic_8.Error_Code_1,1) ,COP(Raw_546xx_Input[391],Mapped_546xx_Communication_Data.I.Diagnostic_8.Error_Code_2,1) ,BTD(Raw_546xx_Input[392],6,Mapped_546xx_Communication_Data.I.Diagnostic_8.Severity,0,2) ];
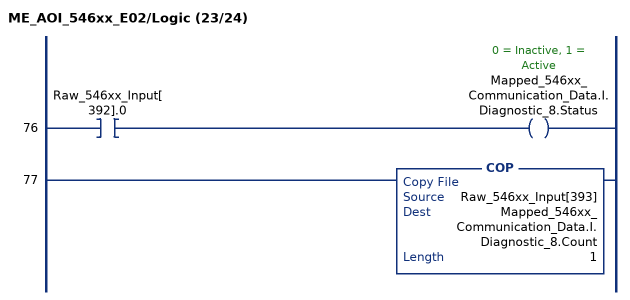
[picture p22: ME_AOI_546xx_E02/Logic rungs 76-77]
   76: XIC(Raw_546xx_Input[392].0)OTE(Mapped_546xx_Communication_Data.I.Diagnostic_8.Status);
   77: COP(Raw_546xx_Input[393],Mapped_546xx_Communication_Data.I.Diagnostic_8.Count,1);
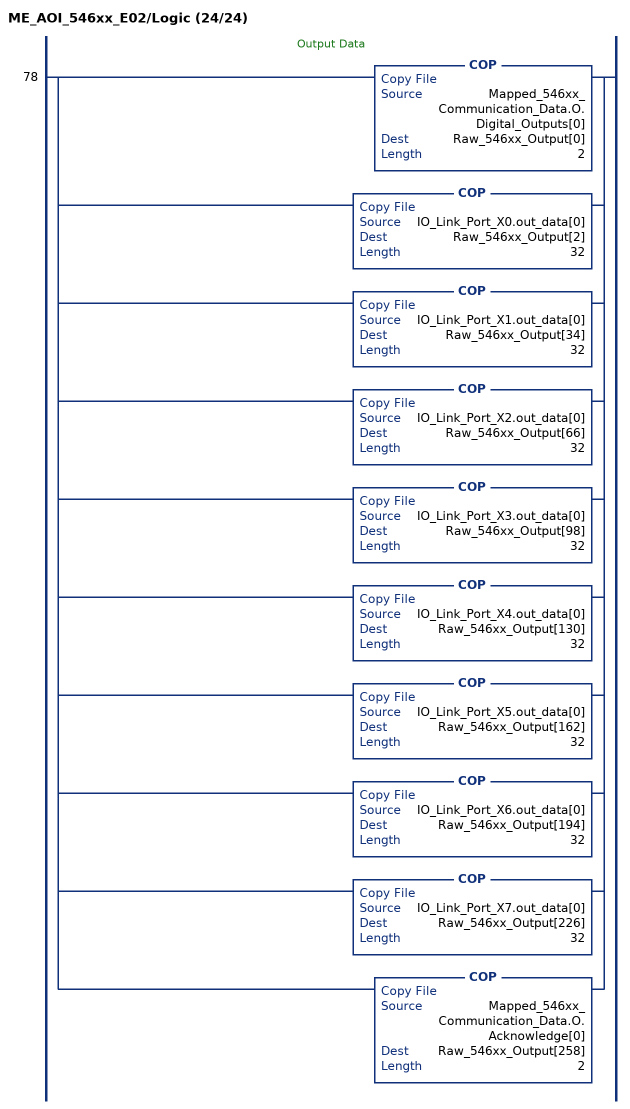
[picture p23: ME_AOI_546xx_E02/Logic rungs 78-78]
   // Output Data
   78: [COP(Mapped_546xx_Communication_Data.O.Digital_Outputs[0],Raw_546xx_Output[0],2) ,COP(IO_Link_Port_X0.out_data[0],Raw_546xx_Output[2],32) ,COP(IO_Link_Port_X1.out_data[0],Raw_546xx_Output[34],32) ,COP(IO_Link_Port_X2.out_data[0],Raw_546xx_Output[66],32) ,COP(IO_Link_Port_X3.out_data[0],Raw_546xx_Output[98],32) ,COP(IO_Link_Port_X4.out_data[0],Raw_546xx_Output[130],32) ,COP(IO_Link_Port_X5.out_data[0],Raw_546xx_Output[162],32) ,COP(IO_Link_Port_X6.out_data[0],Raw_546xx_Output[194],32) ,COP(IO_Link_Port_X7.out_data[0],Raw_546xx_Output[226],32) ,COP(Mapped_546xx_Communication_Data.O.Acknowledge[0],Raw_546xx_Output[258],2) ];
END_ROUTINE
END_ADD_ON_INSTRUCTION
